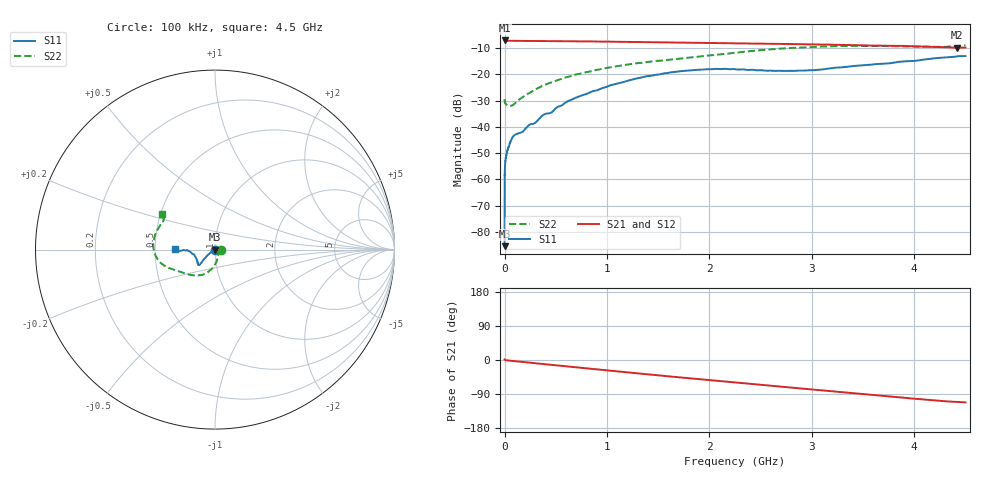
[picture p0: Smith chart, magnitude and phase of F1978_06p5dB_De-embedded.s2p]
! Integrated Device Technology
! Corporate Headquarters
! 6024 Silver Creek Valley Road
! San Jose, CA 95138  USA
! Phone:  1-408-284-8200
! Toll Free:  1-800-223-1366
! Webpage:  http://www.idt.com/
! Timing and RF Division
! 515 Groton Road, Suite 102
! Westford, MA 01886-6024
! Device:  F1978
! Description: 6-bit, 75 ohm, 0.5 dB Digital Step Attenuator
! Frequency:  5.0 MHz -  3.00 GHz
! Package:  4x4 mm QFN Plastic Package: 20 pin
! Ports:  2 RF, 11 DC
!  Pin  1  = D5 (16 dB)
!  Pin  2  = RF1  =  Port 1
!  Pin  3  = Serial Data In (DATA)
!  Pin  4  = Serial Clock (CLK)
!  Pin  5  = Serial Latch Enable (LE)
!  Pin  6  = VDD
!  Pin  7  = NC
!  Pin  8  = NC
!  Pin  9  = NC
!  Pin 10  = GND
!  Pin 11  = GND
!  Pin 12  = NC
!  Pin 13  = VMODE
!  Pin 14  = RF2  =  Port 2
!  Pin 15  = D4 (8 dB)
!  Pin 16  = D3 (4 dB)
!  Pin 17  = D2 (2 dB)
!  Pin 18  = NC
!  Pin 19  = D1 (1 dB)
!  Pin 20  = D0 (0.5 dB)
! State:  13
! Atten State:  6.5 dB
! Voltage:  +3.30 Volts
! Current:  0.560 mA
! Data:  The device was measured on a F1975 evaluation board which has
!  individual transmission lines to the RF pins.  Data was collected
!  using a calibrated network analyzer.  The evaluation board was
!  de-embedded using Automatic Fixture Removal (AFR).
!  The reference plane is the edge of the package pin.
! Misc:
!  Action Tracker AT0416
! Date Measured:  2018-02-08
! Date:  2018-03-26  MJV
! Note:
!  Integrated Device Technology supplies this data as a sample of measured
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# GHz S dB R 75
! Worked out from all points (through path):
!   291 points, 100 kHz to 4.5 GHz, reference 75 ohm
!   highest |S21| = -7.17 dB at 100 kHz (marker M1); lowest = -9.9 dB at 4.42 GHz (marker M2)
!   group delay of S21, straight-line fit = 70.6 ps
!   lowest |S11| = -85.4 dB at 100 kHz (marker M3), VSWR 1.00, Z = 75 + j0.00781 ohm
!   |S11| at or under -10 dB: start of sweep to end of sweep
!   |S22| runs from -32.0 to -9.0 dB; largest |S21 - S12| = 0.00021
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0.0001  -85.37 104.9  -7.17 1.2  -7.18 1.2  -29.47 -0.3
0.0002  -68.96 -126.9  -7.18 1.1  -7.18 1.2  -29.65 -1.3
0.0003  -64.96 -138.1  -7.19 1.1  -7.19 1.1  -29.88 -2.0
0.0005  -59.10 -150.6  -7.20 1.1  -7.20 1.1  -30.06 -2.4
0.0007  -60.51 -156.9  -7.20 1.0  -7.21 1.0  -30.24 -2.8
0.0008  -58.30 -148.3  -7.21 1.0  -7.21 1.0  -30.31 -2.5
0.0009  -58.78 -144.8  -7.21 1.0  -7.21 1.0  -30.38 -2.5
0.002  -56.15 -159.4  -7.22 0.8  -7.22 0.8  -30.66 -2.8
0.007  -53.02 -152.8  -7.24 0.0  -7.24 -0.0  -31.10 -7.2
0.029  -48.58 -154.5  -7.27 -1.1  -7.27 -1.1  -31.78 -17.7
0.08  -43.78 -144.4  -7.31 -2.5  -7.30 -2.5  -31.77 -39.0
0.18  -41.80 -137.2  -7.35 -5.3  -7.35 -5.3  -28.64 -61.1
0.36  -36.04 -143.4  -7.40 -10.2  -7.40 -10.2  -24.60 -78.3
0.76  -27.98 -143.3  -7.52 -20.9  -7.52 -20.9  -19.56 -98.2
1.08  -23.74 -140.3  -7.63 -29.5  -7.63 -29.5  -17.04 -110.4
1.52  -20.01 -136.2  -7.84 -40.9  -7.84 -40.9  -14.87 -127.3
1.88  -18.33 -135.7  -8.06 -50.0  -8.05 -50.0  -13.37 -141.8
2.26  -18.13 -140.0  -8.24 -59.4  -8.24 -59.4  -11.81 -154.3
3.02  -18.46 -165.7  -8.68 -78.2  -8.68 -78.2  -9.62 -173.2
3.76  -15.86 -178.3  -9.18 -95.7  -9.18 -95.7  -9.33 164.4
4.42  -13.20 -178.6  -9.91 -110.7  -9.91 -110.7  -9.29 147.6
4.5  -13.11 179.2  -9.89 -112.0  -9.88 -112.0  -9.05 146.2
